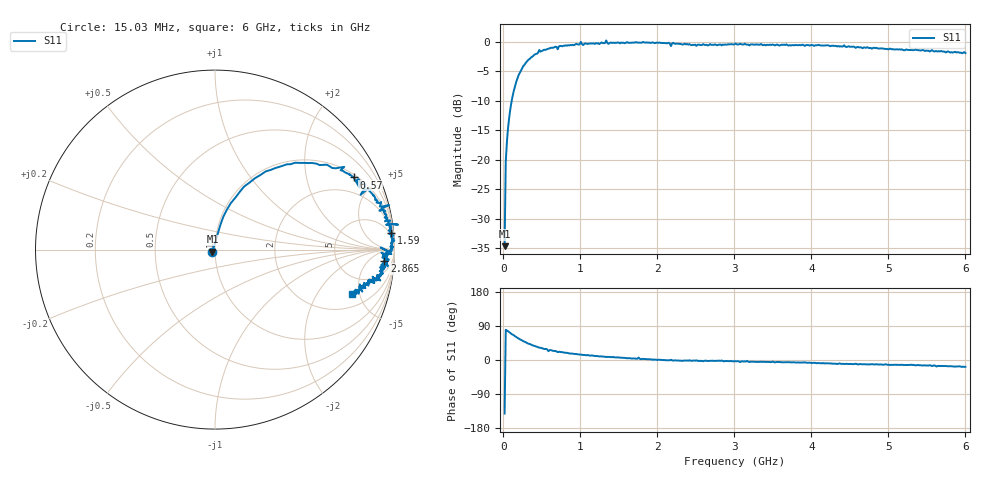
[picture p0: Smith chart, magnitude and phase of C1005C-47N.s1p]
!	Network	Analyzer	HP8753E.07.74:	Oct	30	2002	Serial	No.	JP38451487
!	Hewlett-Packard
!	7	Sep	2009	9:09:26
!	Frequency	S11
#	HZ	S	RI	R	50
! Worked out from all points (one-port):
!   400 points, 15.03 MHz to 6 GHz, reference 50 ohm
!   lowest |S11| = -34.6 dB at 15.03 MHz (marker M1), VSWR 1.04, Z = 48.6 - j1.13 ohm
!   |S11| at or under -10 dB: start of sweep to 106.9 MHz
!   S11 on the Smith chart (normalised r, x): 15.03 MHz: 0.97, -0.02; 570 MHz: 1.13, +3.76; 1.59 GHz: 4, +21; 2.865 GHz: 15, -17; 6 GHz: 3.03, -4.27
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1.502992e7  -0.0145 -0.0116
3.002985e7  0.0172 0.0955
6.00297e7  0.046 0.182
1.200294e8  0.138 0.322
2.850286e8  0.446 0.484
4.650277e8  0.72 0.461
5.700272e8  0.772 0.402
5.850271e8  0.805 0.346
6.150269e8  0.801 0.392
7.050265e8  0.811 0.305
7.650262e8  0.859 0.328
1.005025e9  0.97 0.248
1.035025e9  0.916 0.216
1.245024e9  0.947 0.157
1.335023e9  1.02 0.139
1.365023e9  0.953 0.139
1.515022e9  0.967 0.106
1.590022e9  0.98 0.091
1.755021e9  0.981 0.11
1.785021e9  0.984 0.0364
2.175019e9  0.923 0.0119
2.265019e9  0.968 -0.0234
2.865016e9  0.943 -0.0624
3.015015e9  0.969 -0.0556
3.765011e9  0.934 -0.0958
4.515007e9  0.897 -0.164
5.265004e9  0.833 -0.193
6e9  0.766 -0.248
